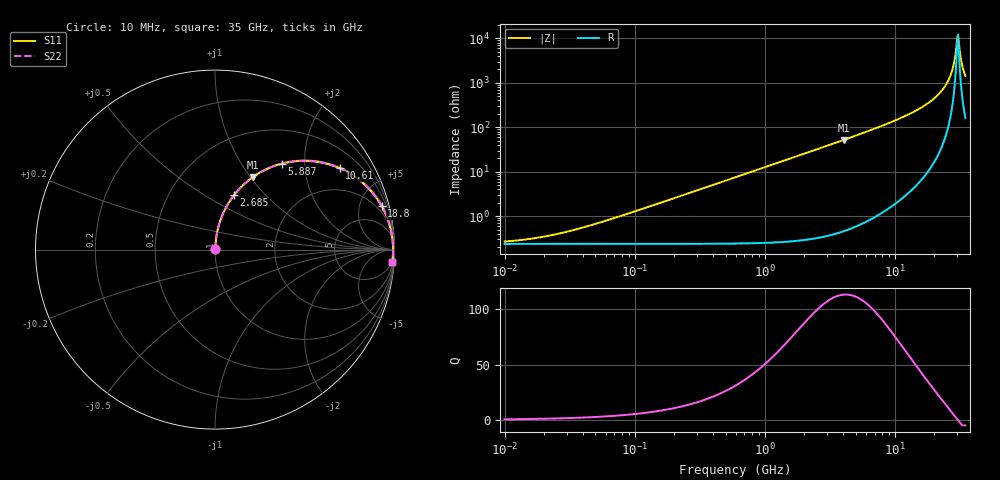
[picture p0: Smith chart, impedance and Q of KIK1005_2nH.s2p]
!version-3
!date-01.2023
!Series
# Hz S RI R 50
!Freq ReS11 ImS11 ReS21 ImS21 ReS12 ImS12 ReS22 ImS22
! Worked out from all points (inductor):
!   500 points, 10 MHz to 35 GHz, reference 50 ohm
!   read as one part in series: L = 2 nH near 57.54 MHz
!   highest Q = 113 at 4.042 GHz (marker M1), where L = 2.04 nH
!   self-resonance near 30.21 GHz
!   S11 on the Smith chart (normalised r, x): 10 MHz: 1.00, +0.00; 2.685 GHz: 1.01, +0.68; 5.887 GHz: 1.01, +1.54; 10.61 GHz: 1.04, +3.03; 18.8 GHz: 1.24, +7.58; 35 GHz: 4, -28
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1e7  0.00237 0.00125  0.9976 -0.00125  0.9976 -0.00125  0.00237 0.00125
1.955222e7  0.00238 0.00245  0.9976 -0.00245  0.9976 -0.00245  0.00238 0.00245
3.949996e7  0.0024 0.00494  0.9976 -0.00494  0.9976 -0.00494  0.0024 0.00494
1.534938e8  0.00274 0.0192  0.9973 -0.0192  0.9973 -0.0192  0.00274 0.0192
5.964653e8  0.00797 0.0742  0.992 -0.0742  0.992 -0.0742  0.00797 0.0742
2.317819e9  0.0814 0.2683  0.9186 -0.2683  0.9186 -0.2683  0.0814 0.2683
2.685348e9  0.106 0.303  0.894 -0.303  0.894 -0.303  0.106 0.303
4.041653e9  0.2129 0.405  0.7871 -0.405  0.7871 -0.405  0.2129 0.405
5.887256e9  0.3723 0.4787  0.6277 -0.4787  0.6277 -0.4787  0.3723 0.4787
9.006867e9  0.6043 0.483  0.3957 -0.483  0.3957 -0.483  0.6043 0.483
1.060711e10  0.6939 0.4539  0.3061 -0.4539  0.3061 -0.4539  0.6939 0.4539
1.447244e10  0.8408 0.356  0.1592 -0.356  0.1592 -0.356  0.8408 0.356
1.880092e10  0.9283 0.2427  0.0717 -0.2427  0.0717 -0.2427  0.9283 0.2427
2.287743e10  0.9694 0.1477  0.0306 -0.1477  0.0306 -0.1477  0.9694 0.1477
2.60751e10  0.9851 0.0819  0.0149 -0.0819  0.0149 -0.0819  0.9851 0.0819
2.783782e10  0.9896 0.0487  0.0104 -0.0487  0.0104 -0.0487  0.9896 0.0487
2.876338e10  0.991 0.032  0.00903 -0.032  0.00903 -0.032  0.991 0.032
2.971971e10  0.9918 0.0152  0.00823 -0.0152  0.00823 -0.0152  0.9918 0.0152
3.070784e10  0.992 -0.00149  0.00798 0.00149  0.00798 0.00149  0.992 -0.00149
3.121416e10  0.9919 -0.00986  0.00807 0.00986  0.00807 0.00986  0.9919 -0.00986
3.33243e10  0.9901 -0.0433  0.00985 0.0433  0.00985 0.0433  0.9901 -0.0433
3.5e10  0.9873 -0.0683  0.0127 0.0683  0.0127 0.0683  0.9873 -0.0683
